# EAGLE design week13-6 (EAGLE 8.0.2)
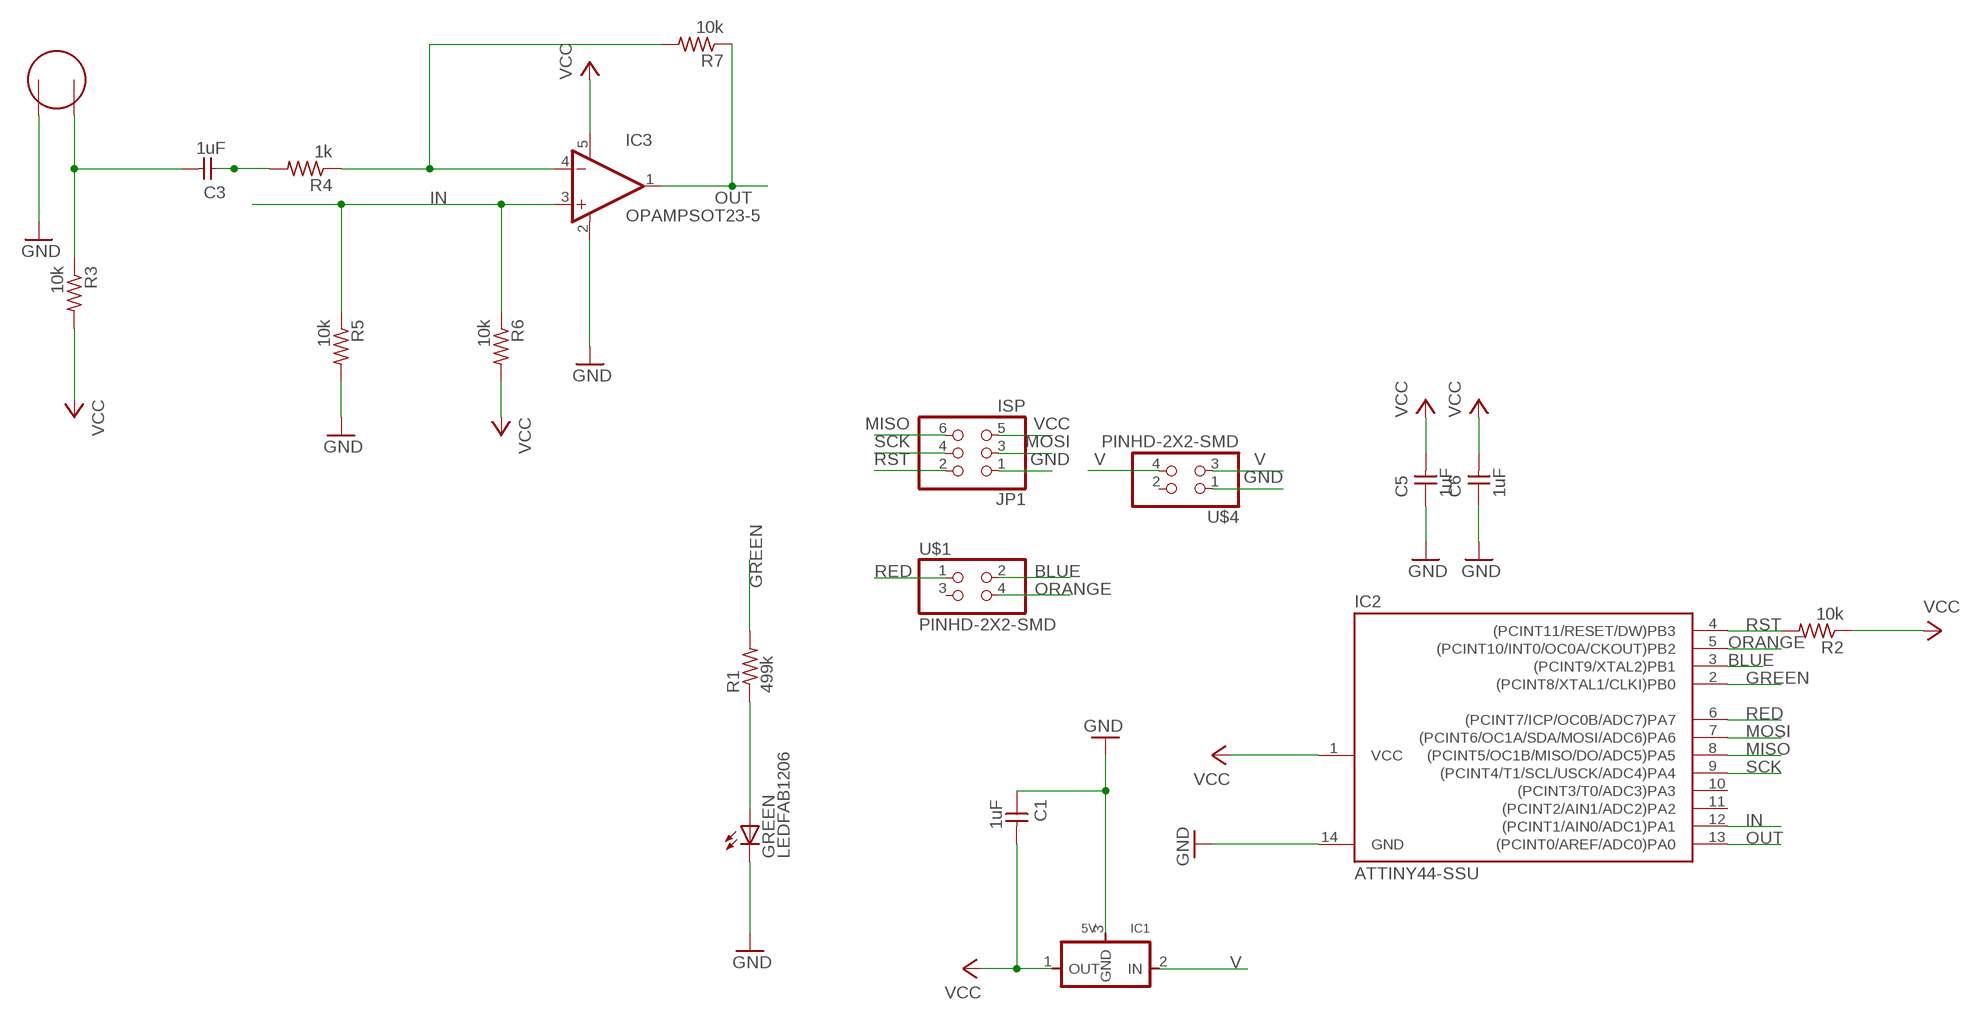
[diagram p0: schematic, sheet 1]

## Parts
C1  1uF  CAP-UNPOLARIZEDFAB  [C1206FAB]
C3  1uF  CAP-UNPOLARIZEDFAB  [C1206FAB]
C5  1uF  CAP-UNPOLARIZEDFAB  [C1206FAB]
C6  1uF  CAP-UNPOLARIZEDFAB  [C1206FAB]
GREEN  LEDFAB1206  [LED1206FAB]
IC1  5V  REGULATORSOT23  [SOT23]
IC2  ATTINY44-SSU  [SOIC14]
IC3  OPAMPSOT23-5  [SOT23-5]
JP1  ISP  PINHD-2X3-SMD  [2X03SMD]
R1  499k  RES-US1206FAB  [R1206FAB]
R2  10k  RES-US1206FAB  [R1206FAB]
R3  10k  RES-US1206FAB  [R1206FAB]
R4  1k  RES-US1206FAB  [R1206FAB]
R5  10k  RES-US1206FAB  [R1206FAB]
R6  10k  RES-US1206FAB  [R1206FAB]
R7  10k  RES-US1206FAB  [R1206FAB]
U$1  PINHD-2X2-SMD  [2X02SMD]
U$2  ELECTRET  [ELECTRET_2742PBJ-A]
U$4  PINHD-2X2-SMD  [2X02SMD]

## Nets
BLUE: IC2.3((PCINT9/XTAL2)PB1) U$1.2
GND: C1.1 C5.1 C6.1 GREEN.2(C) IC1.3(GND) IC2.14(GND) IC3.2(V-) JP1.1 R5.2 U$2.P$1 U$4.1
GREEN: IC2.2((PCINT8/XTAL1/CLKI)PB0) R1.2
IN: IC2.12((PCINT1/AIN0/ADC1)PA1) IC3.3(+IN) R5.1 R6.1
MISO: IC2.8((PCINT5/OC1B/MISO/DO/ADC5)PA5) JP1.6
MOSI: IC2.7((PCINT6/OC1A/SDA/MOSI/ADC6)PA6) JP1.3
N$1: GREEN.1(A) R1.1
N$2: IC3.4(-IN) R4.1 R7.2
N$5: C3.1 R4.2
N$6: C3.2 R3.1 U$2.P$2
ORANGE: IC2.5((PCINT10/INT0/OC0A/CKOUT)PB2) U$1.4
OUT: IC2.13((PCINT0/AREF/ADC0)PA0) IC3.1(OUT) R7.1
RED: IC2.6((PCINT7/ICP/OC0B/ADC7)PA7) U$1.1
RST: IC2.4((PCINT11/RESET/DW)PB3) JP1.2 R2.2
SCK: IC2.9((PCINT4/T1/SCL/USCK/ADC4)PA4) JP1.4
V: IC1.2(IN) U$4.3 U$4.4
VCC: C1.2 C5.2 C6.2 IC1.1(OUT) IC2.1(VCC) IC3.5(V+) JP1.5 R2.1 R3.2 R6.2
Unconnected: IC2.10((PCINT3/T0/ADC3)PA3) IC2.11((PCINT2/AIN1/ADC2)PA2) U$1.3 U$4.2

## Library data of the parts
C1 C3 C5 C6 = fab:CAP-UNPOLARIZED
GREEN = fab:LED: LED
IC1 = fab:REGULATOR
IC2 = fab:ATTINY44
IC3 = fab:OPAMP: Rail-to-Rail Operational Amplifiers Single-Supply, MicroAmplifier(TM) Series
JP1 = fab:PINHD-2X3-SMD: PIN HEADER
R1-R7 = fab:RES-US: Resistor (US Symbol)
U$1 U$4 = fab:PINHD-2X2-SMD
U$2 = fab:ELECTRET

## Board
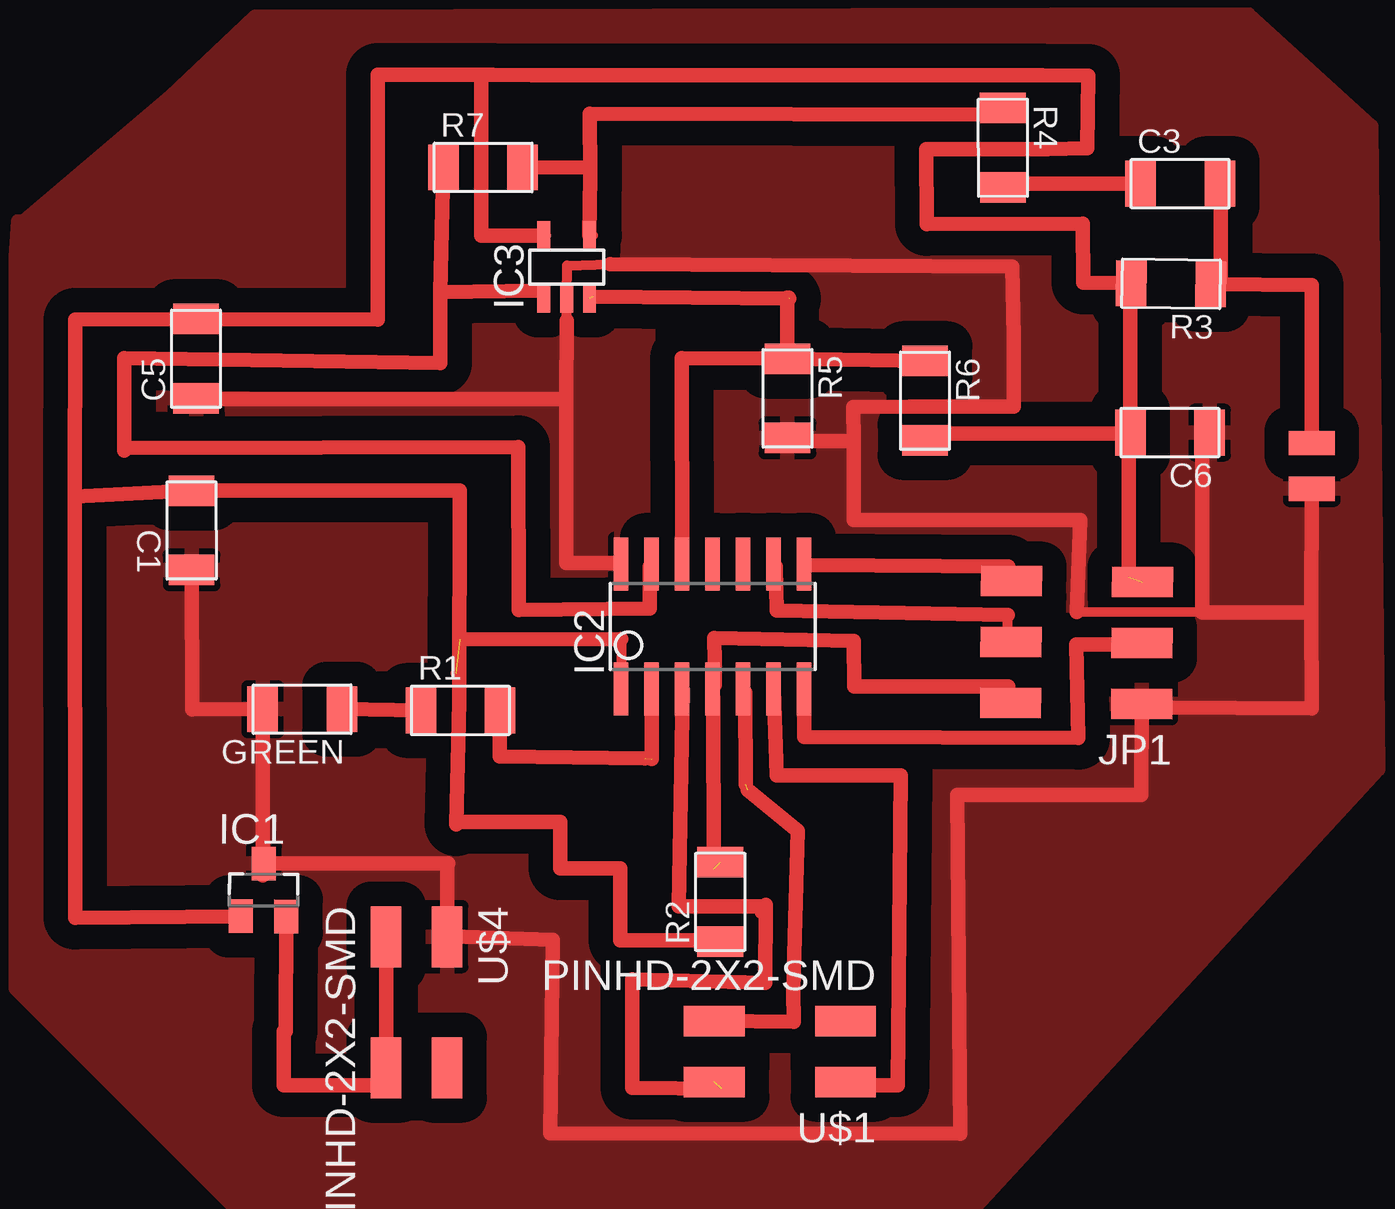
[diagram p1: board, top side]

No outline drawn. Coordinates in mm, seen from the top.
Copper layers (1*16): Top 0.035mm / dielectric 1.5mm / Bottom 0.035mm
Design rules "default *": minimum track width 16mil, minimum drill 24mil, track to track 16mil, track to pad 16mil, pad to pad 16mil, via to via 16mil, smd to smd 8mil, copper to edge 40mil, drill to drill 8mil, minimum pad ring 10mil, minimum via ring 8mil, stop-mask expansion 4mil, vias tented up to drill 0mil, thermal gap 10mil

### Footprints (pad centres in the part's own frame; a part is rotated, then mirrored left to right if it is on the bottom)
C1206FAB = smd 1.27 x 1.905: 1 -1.651,0; 2 1.651,0
LED1206FAB = smd 1.27 x 1.905: 1 -1.651,0; 2 1.651,0
SOT23 = smd 1 x 1.4: 1 -0.95,-1.1; 2 0.95,-1.1; 3 0,1.1
SOIC14 = smd 0.61 x 2.21: 1 -3.81,-2.603; 2 -2.54,-2.603; 3 -1.27,-2.603; 4 0,-2.603; 5 1.27,-2.603; 6 2.54,-2.603; 7 3.81,-2.603; 8 3.81,2.603; 9 2.54,2.603; 10 1.27,2.603; 11 0,2.603; 12 -1.27,2.603; 13 -2.54,2.603; 14 -3.81,2.603
SOT23-5 = smd 0.533 x 1.194: 1 -0.95,-1.306; 2 0,-1.306; 3 0.95,-1.306; 4 0.95,1.306; 5 -0.95,1.306
2X03SMD = smd 2.54 x 1.27: 1 -2.54,2.54; 2 2.92,2.54; 3 -2.54,0; 4 2.92,0; 5 -2.54,-2.54; 6 2.92,-2.54
R1206FAB = smd 1.27 x 1.905: 1 -1.651,0; 2 1.651,0
2X02SMD = smd 2.54 x 1.27: 1 -2.54,1.27; 2 2.92,1.27; 3 -2.54,-1.27; 4 2.92,-1.27
ELECTRET_2742PBJ-A = smd 1.016 x 1.905: P$1 -0.953,0; P$2 0.953,0

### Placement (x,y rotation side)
C1  39.48,55.81 90.1 top
C3  80.67,70.26 0 top
C5  39.66,62.96 90 top
C6  80.24,59.88 180 top
GREEN  44.09,48.35 180 top
IC1  42.48,40.82 359.8 top
IC2  61.19,51.79 0 top
IC3  55.1,66.78 0 top
JP1  76.54,51.13 179.6 top
R1  50.68,48.3 0 top
R2  61.5,40.32 90 top
R3  80.29,66.08 179.3 top
R4  73.29,71.76 270.1 top
R5  64.31,61.31 270 top
R6  70.04,61.21 270 top
R7  51.62,70.93 0 top
U$1  64.19,34.09 180 top
U$2  86.15,58.49 90 top
U$4  48.85,36.33 270 top

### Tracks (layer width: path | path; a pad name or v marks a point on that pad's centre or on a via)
BLUE  (1 unrouted)
  Top 0.406: 59.94,49.17 IC2.3
  Top 0.61: 59.94,49.17 59.79,40.13 63.31,40.14 63.23,39.9 63.4,40.2 63.38,36.94 57.85,37.1 57.85,32.58 61.57,32.53
GND
  Top 0.406: 55.11,64.55 IC3.2 55.09,65.56 55.11,66.84 56.93,66.9 | 57.31,54.45 IC2.14 | 39.69,61.28 C5.1 | C1.1 39.53,54.13 | 81.6,59.85 C6.1 | 79.22,48.58 JP1.1 79.85,48.42 | 69.41,60.96 68.9,60.96 | R5.2 64.84,59.66 64.84,59.52 | 81.6,52.39 76.37,52.41
  Top 0.61: 55.09,61.28 55.09,54.45 57.31,54.45 | 55.09,61.28 55.11,64.55 | 55.09,61.28 39.69,61.28 | 86.13,52.39 81.6,52.39 81.6,59.85 | 86.13,52.39 U$2.P$1 | 50.28,38.87 54.53,38.74 54.42,30.68 71.5,30.65 71.37,44.78 79.05,44.78 JP1.1 | 76.37,52.41 76.51,56.23 67.06,56.23 67.06,59.52 | 67.06,59.52 64.84,59.52 | 56.93,66.9 73.68,66.79 73.73,63.86 73.73,60.96 69.41,60.96 67.04,60.94 67.06,59.52 | 86.13,52.39 86.15,48.38 79.85,48.42 | C1.1 39.51,48.34 GREEN.2 42.45,41.42 | IC1.3 50.16,41.93 50.12,41.93 U$4.1
  pour Top (isolate 1.016): 32.38,68.58 38.61,73.89 42.13,77.23 83.5,77.32 88.63,72.66 88.91,45.83 71.66,27.07 41.81,27.07 32.15,36.73 32.15,67.2 32.26,68.7 32.26,68.47
GREEN  (1 unrouted)
  Top 0.406: 52.31,47.86 52.7,47.47 | 52.31,47.86 52.07,48.1 R1.2 | 58.58,48.1 58.58,49.05 IC2.2 | 58.65,46.29 58.66,48.76 | 52.33,47.86 52.31,47.86
  Top 0.61: IC2.2 58.65,46.29 | 58.35,46.3 52.33,46.38 52.33,47.86
IN  (2 unrouted)
  Top 0.406: R6.1 70.01,62.87 | 56.22,65.55 56.98,65.46
  Top 0.61: R5.1 R6.1 | R5.1 59.9,62.99 IC2.12 | 64.36,65.51 64.31,65.51 R5.1 | 64.38,65.46 56.22,65.55
MISO
  Top 0.406: 73.52,54.31 73.5,53.82 JP1.6 | 65.16,54.36 IC2.8
  Top 0.61: 73.52,54.31 65.16,54.36
MOSI
  Top 0.406: 65.09,49.05 IC2.7 | JP1.3 79.06,50.96 78.65,50.96 78.65,51.04
  Top 0.61: IC2.7 65.01,47.19 76.42,47.15 76.35,51.04 78.65,51.04
N$1
  Top 0.61: GREEN.1 R1.1
N$2
  Top 0.406: 56.04,68.1 IC3.4 56.2,68.1 | 53.34,70.8 R7.2 | 72.87,73.03 72.96,73.12 73.18,73.34 R4.1 | 56.1,70.94 56.09,70.58
  Top 0.61: R7.2 56.1,70.94 | 56.04,68.1 56.09,70.58 56.06,73.18 72.96,73.12
N$5
  Top 0.406: 73.66,70.48 73.34,70.17 R4.2 73.44,70.25
  Top 0.61: 73.44,70.25 C3.1
N$6
  Top 0.406: 82.37,66.04 82.07,66.04 R3.1 | C3.2 82.37,70.2
  Top 0.61: 82.37,70.2 82.37,66.04 | R3.1 86.15,66.03 U$2.P$2
ORANGE  (1 unrouted)
  Top 0.406: 62.55,49.05 IC2.5
  Top 0.61: 62.57,45.21 62.55,49.05 | 62.66,44.98 64.74,43.27 64.55,36.64 64.57,35.32 U$1.4
OUT
  Top 0.406: 53.91,65.79 54.13,65.56 IC3.1 | R7.1 50.01,70.8 50.01,69.69 49.85,69.69 | 58.58,54.29 IC2.13
  Top 0.61: 58.58,54.29 58.58,52.55 53.11,52.48 53.08,59.29 36.77,59.23 36.68,59.14 36.68,62.98 49.84,62.79 49.84,65.74 | R7.1 49.84,65.74 | 49.84,65.74 53.91,65.79
RED
  Top 0.61: IC2.6 63.74,49.19 63.87,45.58 69.04,45.58 68.91,32.68 66.72,32.68 U$1.1
RST  (1 unrouted)
  Top 0.406: 61.22,48.83 61.28,49.05 IC2.4 61.28,49.37 | 73.51,49.3 73.5,48.74 JP1.2
  Top 0.61: 61.22,48.83 61.24,41.69 | 73.51,49.3 67.08,49.3 67.07,51.2 61.25,51.32 61.28,50.32 61.28,49.37
SCK
  Top 0.406: 73.48,52.28 73.5,51.28 JP1.4 | 63.82,54.29 IC2.9
  Top 0.61: 63.82,54.29 63.86,52.46 73.48,52.28
V
  Top 0.61: IC1.2 43.39,34.92 43.33,34.92 43.33,32.66 47.58,32.66 U$4.4 U$4.3
VCC  (2 unrouted)
  Top 0.406: 70.33,59.85 70.17,59.69 R6.2 | 78.11,59.85 C6.2 | 78.58,60.01 78.26,60.01 C6.2 | 78.58,66.04 R3.2 78.42,66.04 | IC3.5 54.13,68.1 | C5.2 39.69,64.77 39.66,64.75 C5.2 | 50.64,48.68 50.64,49.85 50.48,49.85 | 57.31,49.21 IC2.1 57.38,51.27 | 39.53,57.31 C1.2 | 39.37,64.29 39.53,64.45 C5.2 | C6.2 78.53,59.83 | 52.02,74.8 51.54,74.8 51.35,74.81 | 50.5,43.56 50.5,43.66
  Top 0.61: 78.11,59.85 70.33,59.85 | 78.58,60.01 78.58,66.04 | 50.5,43.56 50.64,48.68 50.66,57.46 C1.2 34.6,57.22 | 50.65,51.26 57.38,51.27 | 78.53,59.83 78.53,53.86 | R3.2 76.64,66.13 76.61,68.59 70.11,68.57 70.1,71.7 75.15,71.7 76.81,71.74 76.84,74.75 74.93,74.77 53.66,74.77 52.02,74.8 47.24,74.8 47.24,64.59 C5.2 34.62,64.6 34.6,57.22 | 34.6,57.22 34.64,39.66 IC1.1 | 51.54,74.8 51.54,68.09 IC3.5 | 50.5,43.66 54.85,43.66 54.85,41.71 57.33,41.71 57.33,38.72 61.5,38.72 R2.1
